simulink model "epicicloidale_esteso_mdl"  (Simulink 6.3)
settings: Solver=ode45  StartTime=0.0  StopTime=0.1  RelTol=1e-3
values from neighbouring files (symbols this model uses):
  b_c = kb*J_c    (= 4.94590955184)    [architetture_epicicloidale.m]    (also in architetture_epicicloidale_cont.m; architetture_epicicloidale_HEV.m = 92.8974810391; architetture_epicicloidale_prova.m; architetture_HEV_controllo.m = 9.28974810391)
  b_r = kb*J_r    (= 218.026030555)    [architetture_epicicloidale.m]    (also in architetture_epicicloidale_cont.m; architetture_epicicloidale_HEV.m; architetture_epicicloidale_prova.m; architetture_HEV_controllo.m = 21.8026030555)
  b_s = kb*J_s    (= 8.12277148259)    [architetture_epicicloidale.m]    (also in architetture_epicicloidale_cont.m; architetture_epicicloidale_HEV.m = 4.94590955184; architetture_epicicloidale_prova.m; architetture_HEV_controllo.m = 0.494590955184)
  b_sc = kb*J_sc    (= 92.8974810391)    [architetture_epicicloidale.m]    (also in architetture_epicicloidale_cont.m; architetture_epicicloidale_prova.m; epicicloidale.m; epicicloidale_da_solo.m)
  d_cs = d0    (= 10)    [architetture_epicicloidale.m]    (also in architetture_epicicloidale_cont.m; architetture_epicicloidale_prova.m; epicicloidale.m; epicicloidale_da_solo.m)
  d_sr = d0    (= 10)    [architetture_epicicloidale.m]    (also in architetture_epicicloidale_cont.m; architetture_epicicloidale_prova.m; epicicloidale.m; epicicloidale_da_solo.m)
  J_c = 1.3*0.5*pi*rho_acc*hc*r_c^4    (= 0.0494590955184)    [architetture_epicicloidale.m]    (also in architetture_epicicloidale_cont.m; architetture_epicicloidale_HEV.m = 0.928974810391; architetture_epicicloidale_prova.m; architetture_HEV_controllo.m = 0.928974810391)
  J_r = 0.5*pi*rho_acc*(hr*r_ri^4 + h_ring*(r_re^4-r_ri^4))    (= 2.18026030555)    [architetture_epicicloidale.m]    (also in architetture_epicicloidale_cont.m; architetture_epicicloidale_HEV.m; architetture_epicicloidale_prova.m; architetture_HEV_controllo.m)
  J_s = Nr_sat*0.5*pi*rho_acc*(hs*r_s^4 + hc*r_s^4)    (= 0.0812277148259)    [architetture_epicicloidale.m]    (also in architetture_epicicloidale_cont.m; architetture_epicicloidale_HEV.m = 0.0494590955184; architetture_epicicloidale_prova.m; architetture_HEV_controllo.m = 0.0494590955184)
  J_sc = Nr_sat*(r_c+r_s)^2*rho_acc*pi*(hs*r_s^2 + hc*r_s^2)    (= 0.928974810391)    [architetture_epicicloidale.m]    (also in architetture_epicicloidale_cont.m; architetture_epicicloidale_prova.m; epicicloidale.m; epicicloidale_da_solo.m)
  K_cs = K0    (= 10000000)    [architetture_epicicloidale.m]    (also in architetture_epicicloidale_cont.m; architetture_epicicloidale_prova.m; epicicloidale.m; epicicloidale_da_solo.m)
  K_sr = K0    (= 10000000)    [architetture_epicicloidale.m]    (also in architetture_epicicloidale_cont.m; architetture_epicicloidale_prova.m; epicicloidale.m; epicicloidale_da_solo.m)
  Nr_sat = 4    [architetture_epicicloidale.m]    (also in architetture_epicicloidale_cont.m; architetture_epicicloidale_HEV.m; architetture_epicicloidale_prova.m; architetture_HEV_controllo.m)
  r_c = r_ri-2*r_s    (= 0.101859163579)    [architetture_epicicloidale.m]    (also in architetture_epicicloidale_cont.m; architetture_epicicloidale_prova.m; epicicloidale.m; epicicloidale_da_solo.m)
  r_ri = xds*Nr/(2*pi)    (= 0.248281711223)    [architetture_epicicloidale.m]    (also in architetture_epicicloidale_cont.m; architetture_epicicloidale_prova.m; epicicloidale.m; epicicloidale_da_solo.m)
  r_s = xds*Ns/(2*pi)    (= 0.0732112738223)    [architetture_epicicloidale.m]    (also in architetture_epicicloidale_cont.m; architetture_epicicloidale_HEV.m = 0.101859163579; architetture_epicicloidale_prova.m; architetture_HEV_controllo.m = 0.101859163579)
  Tau_c = 0*N*metri    (= 0)    [architetture_epicicloidale.m]    (also in architetture_epicicloidale_cont.m; architetture_epicicloidale_prova.m; epicicloidale.m; epicicloidale_confronto_statico_elastico.m = 10)
  Tau_r = 0*N*metri    (= 0)    [architetture_epicicloidale.m]    (also in architetture_epicicloidale_cont.m; architetture_epicicloidale_prova.m; epicicloidale.m; epicicloidale_confronto_statico_elastico.m = 20)
  Tau_sc = 200*N*metri    (= 200)    [architetture_epicicloidale.m]    (also in architetture_epicicloidale_cont.m = 50; architetture_epicicloidale_prova.m = 50; epicicloidale.m = 4; epicicloidale_da_solo.m = 4)
  Tc = 0.05*ms    (= 5e-05)    [architetture_epicicloidale.m]    (also in architetture_epicicloidale_cont.m; architetture_epicicloidale_HEV.m; architetture_epicicloidale_prova.m; architetture_HEV_controllo.m)
  Wc_0 = 0*0.1*rad/secondo    (= 0)    [architetture_epicicloidale.m]    (also in architetture_epicicloidale_cont.m; architetture_epicicloidale_HEV.m; architetture_epicicloidale_prova.m; Confronto_CVT_EMR.m)
  Wr_0 = Sys1.C(3,:)*[Wc_0; Wsc_0]    [architetture_epicicloidale.m]    (also in Confronto_CVT_EMR.m = 0; epicicloidale.m; epicicloidale_confronto_statico_elastico.m = [-r_s/r_r, 1+r_s/r_r]*[Ws_0; Wc_0]; epicicloidale_da_solo.m = [ -1/r_ri*r_c, (r_c+r_ri)/r_ri]*[Wc_0; Wsc_0])
  Wsc_0 = -0*0.2*rad/secondo    (= 0)    [architetture_epicicloidale.m]    (also in architetture_epicicloidale_cont.m; architetture_epicicloidale_HEV.m; architetture_epicicloidale_prova.m; epicicloidale.m = -0.2)

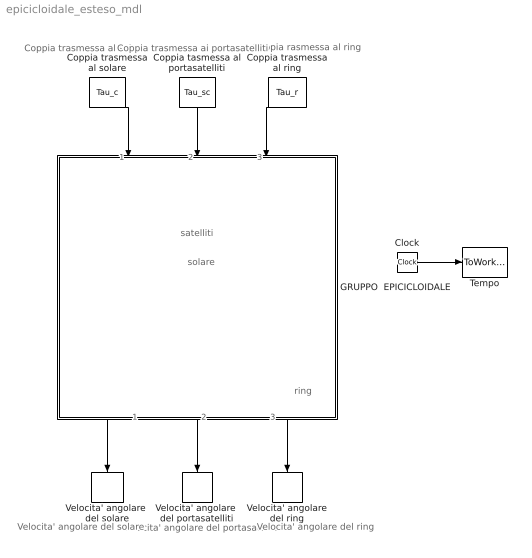
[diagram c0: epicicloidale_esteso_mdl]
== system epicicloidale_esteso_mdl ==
  note: solare
  note: satelliti
  note: ring
  note: Velocita' angolare del portasatelliti
  note: Velocita' angolare del ring
  note: Velocita' angolare del solare
  note: Coppia rasmessa al ring
  note: Coppia trasmessa al solare
  note: Coppia trasmessa ai portasatelliti
  Clock : Clock
  Coppia tasmessa al portasatelliti : Constant  Orientation=down  Value=Tau_sc
  Coppia trasmessa al ring : Constant  Orientation=down  Value=Tau_r
  Coppia trasmessa al solare : Constant  Orientation=down  Value=Tau_c
  GRUPPO  EPICICLOIDALE : Subsystem  Orientation=down  mask(POG Gruppo epicicloidale){Par_solare=[J_c, b_c, r_c], Par_satelliti=[J_s, J_sc, b_s, b_sc, r_s, Nr_sat], Par_ring=[J_r, b_r, r_ri], Solare_Satelliti=[K_cs, d_cs], Satelliti_Ring=[K_sr, d_sr], Cond_in=[Wc_0, Wsc_0, Wr_0]}
      mask prompts: Par_solare "Parametri Solare: [J_c, b_c, r_c]-->[kg*m^2,N*m*s/rad,m]"; Par_satelliti "Parametri Satelliti: [J_s, J_sc, b_s, b_sc, r_s, Nr_sat]-->[kg*m^2,N*m*s/rad,m]"; Par_ring "Parametri Ring: [J_r, b_r, r_ri]-->[kg*m^2,N*m*s/rad,m,m]"; Solare_Satelliti "Solare-Satelliti: [K_cs, d_cs]-->[N/m,N*m*s/rad]"; Satelliti_Ring "Satelliti-Ring: [K_sr, d_sr]-->[N/m,N*m*s/rad]"; Cond_in "Condizioni iniziali: [Wc_0,  Wsc_0,  Wr_0]-->[rad/s]"
      mask help: Gruppo epicicloidale: [J_c, J_s, J_r, J_sc]= Inerzie di: solare, satelliti, ring, solare-ssatelliti; [b_c, b_s, b_r]= Attriti di: solare, satelliti, ring; [r_c, r_s, r_ri, r_re]= Raggi di: solare, satelliti, ring(interno ed esterno); [Nr_sat]= Numero Satelliti; [K_cs, K_sr]= Elasticita' tra solare-satelliti e tra satelliti-ring; [b_sc]= Attriti tra solare-satelliti; [d_cs, d_sr]= Elementi della matrice D; [Wc_0, Wsc_0, Wr_0]=Velocita' iniziali di solare, satelliti, portasatelliti, ring;
      mask init:
      | J_c=double(Par_solare(1));          
      | b_c=double(Par_solare(2));            
      | r_c=double(Par_solare(3));           
      | %
      | J_s=double(Par_satelliti(1));            
      | J_sc=double(Par_satelliti(2));            
      | b_s=double(Par_satelliti(3));            
      | b_sc=double(Par_satelliti(4));            
      | r_s=double(Par_satelliti(5));            
      | Nr_sat=double(Par_satelliti(6));           
      | %
      | J_r=double(Par_ring(1));             
      | b_r=double(Par_ring(2));            
      | r_ri=double(Par_ring(3));                  
      | %
      | K_cs=double(Solare_Satelliti(1));
      | d_cs=double(Solare_Satelliti(2));
      | %
      | K_sr=double(Satelliti_Ring(1));
      | d_sr=double(Satelliti_Ring(2));
      | %
      | %%%%%%%%%%%%%%%%%%%%%%%%%%%%%
      | %   Modello esteso 
      | %%%%%%%%%%%%%%%%%%%%%%%%%%%%%
      | Wc_0=double(Cond_in(1));
      | Wsc_0=double(Cond_in(2));
      | Wr_0=double(Cond_in(3));
      | Ws_0=r_c*(Wsc_0-Wc_0)/r_s;
      | Ws_sc_0=[Ws_0 Wsc_0];
      | %
      | Rsc=[-r_s; r_c];
      | B_Tsc=[0;1];       % Matrice di selezione
      | JJs0=diag([J_s, J_sc]);
      | Bs0=diag([b_s, b_sc]);
      | Rsr=[r_s r_ri];
  Tempo : ToWorkspace  VariableName=t  SampleTime=Tc  SaveFormat=Array
  Velocita' angolare del ring : ToWorkspace  VariableName=W_r  SampleTime=Tc  SaveFormat=Array
  Velocita' angolare  del portasatelliti : ToWorkspace  VariableName=W_sc  SampleTime=Tc  SaveFormat=Array
  Velocita' angolare  del solare : ToWorkspace  VariableName=W_c  SampleTime=Tc  SaveFormat=Array
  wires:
  Clock/1 -> Tempo/1
  Coppia trasmessa al ring/1 -> GRUPPO  EPICICLOIDALE/3(Tau_r)
  Coppia trasmessa al solare/1 -> GRUPPO  EPICICLOIDALE/1(Tau_c)
  GRUPPO  EPICICLOIDALE/2("[w_sc]") -> Velocita' angolare  del portasatelliti/1
  GRUPPO  EPICICLOIDALE/3(w_r) -> Velocita' angolare del ring/1
  Coppia tasmessa al portasatelliti/1 -> GRUPPO  EPICICLOIDALE/2("[Tau_sc]")
  GRUPPO  EPICICLOIDALE/1(w_c) -> Velocita' angolare  del solare/1

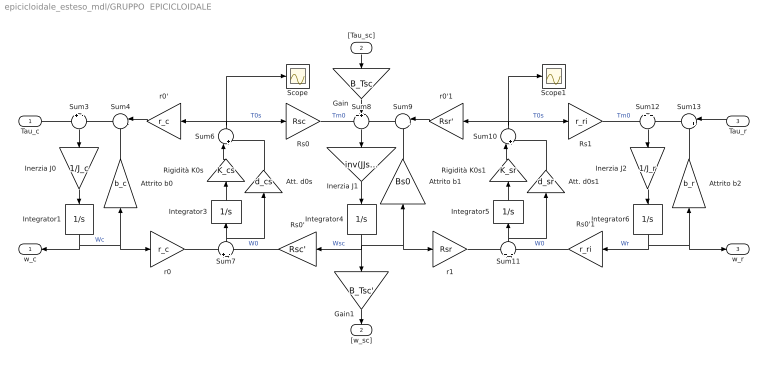
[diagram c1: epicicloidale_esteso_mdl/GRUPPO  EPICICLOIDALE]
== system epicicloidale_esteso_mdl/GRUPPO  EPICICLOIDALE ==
  Tau_c : Inport
  "[Tau_sc]" : Inport  Orientation=down  Port=2
  Tau_r : Inport  Orientation=left  Port=3
  Att. d0s : Gain  Orientation=up  Gain=d_cs
  Att. d0s1 : Gain  Orientation=up  Gain=d_sr
  Attrito b0 : Gain  Orientation=up  Gain=b_c
  Attrito b1 : Gain  Orientation=up  Gain=Bs0  Multiplication=Matrix(K*u)
  Attrito b2 : Gain  Orientation=up  Gain=b_r
  Gain : Gain  Orientation=down  Gain=B_Tsc  Multiplication=Matrix(K*u)
  Gain1 : Gain  Orientation=down  Gain=B_Tsc'  Multiplication=Matrix(K*u)
  Inerzia J0 : Gain  Orientation=down  Gain=1/J_c
  Inerzia J1 : Gain  Orientation=down  Gain=inv(JJs0)  Multiplication=Matrix(K*u)
  Inerzia J2 : Gain  Orientation=down  Gain=1/J_r
  Integrator1 : Integrator  Orientation=down  InitialCondition=Wc_0  LowerSaturationLimit=0
  Integrator3 : Integrator  Orientation=up
  Integrator4 : Integrator  Orientation=down  InitialCondition=Ws_sc_0  LowerSaturationLimit=0
  Integrator5 : Integrator  Orientation=up
  Integrator6 : Integrator  Orientation=down  InitialCondition=Wr_0  LowerSaturationLimit=0
  Rigidità K0s : Gain  Orientation=up  Gain=K_cs
  Rigidità K0s1 : Gain  Orientation=up  Gain=K_sr
  Rs0 : Gain  Gain=Rsc  Multiplication=Matrix(K*u)
  Rs0' : Gain  Orientation=left  Gain=Rsc'  Multiplication=Matrix(K*u)
  Rs0'1 : Gain  Orientation=left  Gain=r_ri
  Rs1 : Gain  Gain=r_ri
  Scope : Scope
  Scope1 : Scope
  Sum10 : Sum  Orientation=up  Inputs=|++
  Sum11 : Sum  Orientation=up  Inputs=+|-
  Sum12 : Sum  Orientation=down  Inputs=+|+
  Sum13 : Sum  Orientation=left  Inputs=|+-
  Sum3 : Sum  Orientation=down  Inputs=+|-
  Sum4 : Sum  Orientation=left  Inputs=|++
  Sum6 : Sum  Orientation=up  Inputs=|++
  Sum7 : Sum  Orientation=up  Inputs=+|-
  Sum8 : Sum  Orientation=down  Inputs=++-
  Sum9 : Sum  Orientation=left  Inputs=|++
  r0 : Gain  Gain=r_c
  r0' : Gain  Orientation=left  Gain=r_c
  r0'1 : Gain  Orientation=left  Gain=Rsr'  Multiplication=Matrix(K*u)
  r1 : Gain  Gain=Rsr  Multiplication=Matrix(K*u)
  w_c : Outport  Orientation=left
  "[w_sc]" : Outport  Orientation=down  Port=2
  w_r : Outport  Port=3
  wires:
  Sum4/1 -> Sum3/2
  Rs0/1 -> Sum8/1  "Tm0"
  Sum9/1 -> Sum8/3
  Sum13/1 -> Sum12/2
  Attrito b2/1 -> Sum13/2
  Integrator6/1 -> Attrito b2/1, w_r/1, Rs0'1/1  "Wr"
  Inerzia J2/1 -> Integrator6/1
  Sum12/1 -> Inerzia J2/1
  Rs1/1 -> Sum12/1  "Tm0"
  r1/1 -> Sum11/1
  Rs0'1/1 -> Sum11/2  "W0"
  Att. d0s1/1 -> Sum10/2
  Rigidità K0s1/1 -> Sum10/1
  Integrator5/1 -> Rigidità K0s1/1
  Sum10/1 -> Rs1/1, r0'1/1, Scope1/1  "T0s"
  Sum11/1 -> Integrator5/1, Att. d0s1/1
  r0'1/1 -> Sum9/1
  Attrito b1/1 -> Sum9/2
  Integrator4/1 -> r1/1, Attrito b1/1, Rs0'/1, Gain1/1  "Wsc"
  Inerzia J1/1 -> Integrator4/1
  Sum8/1 -> Inerzia J1/1
  r0/1 -> Sum7/1
  Rs0'/1 -> Sum7/2  "W0"
  Att. d0s/1 -> Sum6/2
  Rigidità K0s/1 -> Sum6/1
  Integrator3/1 -> Rigidità K0s/1
  Sum6/1 -> r0'/1, Rs0/1, Scope/1  "T0s"
  Sum7/1 -> Att. d0s/1, Integrator3/1
  r0'/1 -> Sum4/1
  Attrito b0/1 -> Sum4/2
  Integrator1/1 -> Attrito b0/1, r0/1, w_c/1  "Wc"
  Inerzia J0/1 -> Integrator1/1
  Sum3/1 -> Inerzia J0/1
  Tau_c/1 -> Sum3/1
  Tau_r/1 -> Sum13/1
  Gain/1 -> Sum8/2
  "[Tau_sc]"/1 -> Gain/1
  Gain1/1 -> "[w_sc]"/1
